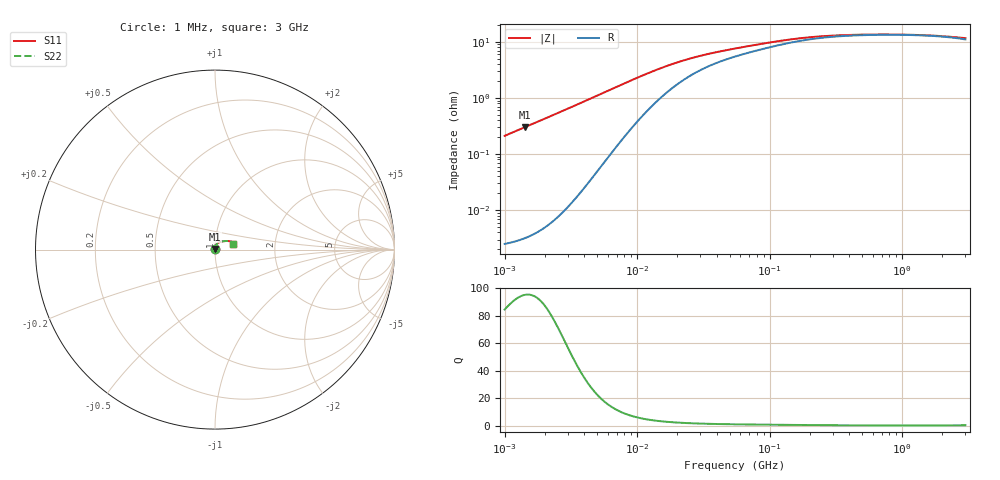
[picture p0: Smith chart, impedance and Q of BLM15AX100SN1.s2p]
! BLM15AX100SN1
# Hz S RI R 50
!Freq.(Hz) S11(Real) S11(Imag) S21(Real) S21(Imag) S12(Real) S12(Imag) S22(Real) S22(Imag)
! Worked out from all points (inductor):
!   401 points, 1 MHz to 3 GHz, reference 50 ohm
!   read as one part in series: L = 33.6 nH near 1.041 MHz
!   highest Q = 95.1 at 1.434 MHz (marker M1), where L = 33.7 nH
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1000000  2.95e-05 0.00211  1 -0.00211  1 -0.00211  2.95e-05 0.00211
1040844  3.03e-05 0.0022  1 -0.0022  1 -0.0022  3.03e-05 0.0022
1433740  4.11e-05 0.00303  1 -0.00303  1 -0.00303  4.11e-05 0.00303
3823119  0.000289 0.00829  0.9997 -0.00829  0.9997 -0.00829  0.000289 0.00829
9223615  0.00345 0.0207  0.9966 -0.0207  0.9966 -0.0207  0.00345 0.0207
1.172775e7  0.00631 0.0259  0.9937 -0.0259  0.9937 -0.0259  0.00631 0.0259
1.461624e7  0.0103 0.031  0.9897 -0.031  0.9897 -0.031  0.0103 0.031
1.973457e7  0.0181 0.0375  0.9819 -0.0375  0.9819 -0.0375  0.0181 0.0375
2.664524e7  0.0281 0.0426  0.9719 -0.0426  0.9719 -0.0426  0.0281 0.0426
3.670325e7  0.0397 0.0457  0.9603 -0.0457  0.9603 -0.0457  0.0397 0.0457
5.477226e7  0.0542 0.0475  0.9458 -0.0475  0.9458 -0.0475  0.0542 0.0475
8.338914e7  0.0695 0.0479  0.9305 -0.0479  0.9305 -0.0479  0.0695 0.0479
1.171891e8  0.0826 0.0464  0.9174 -0.0464  0.9174 -0.0464  0.0826 0.0464
1.582265e8  0.0937 0.0429  0.9063 -0.0429  0.9063 -0.0429  0.0937 0.0429
2.094008e8  0.1026 0.038  0.8974 -0.038  0.8974 -0.038  0.1026 0.038
2.771263e8  0.1093 0.0322  0.8907 -0.0322  0.8907 -0.0322  0.1093 0.0322
3.817355e8  0.1143 0.026  0.8857 -0.026  0.8857 -0.026  0.1143 0.026
8.005644e8  0.1181 0.0165  0.8819 -0.0165  0.8819 -0.0165  0.1181 0.0165
1.147801e9  0.1171 0.015  0.8829 -0.015  0.8829 -0.015  0.1171 0.015
1.581072e9  0.1143 0.016  0.8857 -0.016  0.8857 -0.016  0.1143 0.016
2.092429e9  0.1099 0.0194  0.8901 -0.0194  0.8901 -0.0194  0.1099 0.0194
3e9  0.1004 0.03  0.8996 -0.03  0.8996 -0.03  0.1004 0.03
